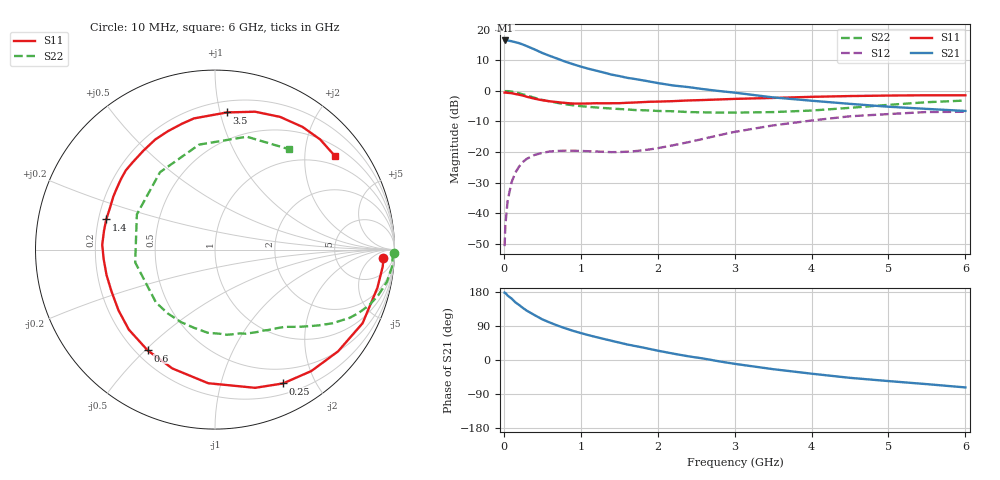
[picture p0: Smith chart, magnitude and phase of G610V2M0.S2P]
! SIEMENS Small Signal Semiconductors
! BFG193
! Si NPN RF Bipolar Junction Transistor in SOT223
! VCE = 10 V  IC = 2 mA
! Common Emitter S-Parameters:  August  1996
# GHz  S  MA  R  50
!  f  S11  S21  S12  S22
! GHz  MAG  ANG  MAG  ANG  MAG  ANG  MAG  ANG
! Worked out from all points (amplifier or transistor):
!   36 points, 10 MHz to 6 GHz, reference 50 ohm
!   highest |S21| = 16.5 dB at 20 MHz (marker M1)
!   |S21| within 3 dB of that: start of sweep to 406 MHz
!   unconditionally stable (mu >= 1): 1.382 GHz to 2.533 GHz
!   at 250 MHz: K = 0.17, MSG = 19.2 dB, |S12| = -23.2 dB
!   at 1.4 GHz: K = 1.02, MAG = 11.9 dB, |S12| = -20.0 dB
!   at 6 GHz: K = 0.94, MSG = 0.1 dB, |S12| = -6.8 dB
!   S11 on the Smith chart (normalised r, x): 10 MHz: 20, -15; 250 MHz: 0.32, -1.58; 600 MHz: 0.25, -0.51; 1.4 GHz: 0.23, +0.13; 3.5 GHz: 0.28, +1.05; 6 GHz: 0.73, +2.71
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0.01  0.9385 -2.7  6.626 177.8  0.0029 92.9  0.9958 -1.1
0.02  0.9394 -5.7  6.674 177.0  0.0065 88.9  0.9905 -2.1
0.05  0.9296 -13.2  6.66 169.9  0.0162 82.7  0.9913 -5.4
0.1  0.919 -26.5  6.489 162.3  0.032 75.2  0.9748 -10.6
0.15  0.8896 -39.6  6.25 152.2  0.0462 67.3  0.9453 -15.5
0.25  0.8363 -63.1  5.71 137.0  0.0693 55.5  0.8757 -23.7
0.3  0.8019 -73.8  5.383 130.0  0.0779 50.7  0.8422 -26.8
0.4  0.7455 -92.9  4.763 118.4  0.09 42.0  0.7713 -32.2
0.5  0.7036 -109.7  4.162 107.3  0.097 34.6  0.7135 -36.3
0.6  0.6754 -123.7  3.727 98.7  0.1025 29.9  0.6715 -39.5
0.7  0.6552 -137.1  3.348 90.7  0.1045 26.0  0.6357 -42.6
0.8  0.6353 -147.8  3.002 83.6  0.1055 22.8  0.6054 -45.3
0.9  0.622 -158.0  2.731 77.0  0.1054 21.2  0.5816 -47.7
1.1  0.6225 -175.0  2.303 65.6  0.1033 19.3  0.5486 -53.7
1.4  0.6288 164.5  1.845 50.7  0.0998 20.5  0.5157 -62.9
1.6  0.6389 152.5  1.639 41.1  0.1015 24.1  0.4986 -70.0
2.2  0.6802 126.0  1.227 16.9  0.1292 34.4  0.4651 -95.0
2.8  0.7247 104.8  0.995 -3.6  0.1891 33.6  0.4424 -126.7
3.5  0.7671 85.0  0.783 -24.2  0.273 19.7  0.4504 -170.9
4.5  0.8235 63.9  0.614 -47.1  0.3848 -4.7  0.5289 125.4
5.5  0.8484 46.4  0.508 -63.7  0.4523 -34.2  0.6535 74.3
6  0.8473 38.2  0.47 -72.4  0.4555 -50.1  0.6958 53.4
